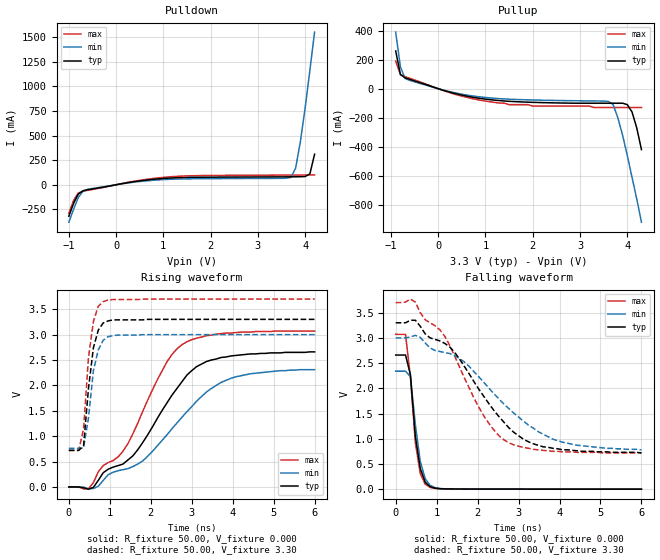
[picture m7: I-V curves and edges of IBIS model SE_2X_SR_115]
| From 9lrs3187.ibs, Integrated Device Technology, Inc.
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|   Model SE_2X_SR_115
[Model]   SE_2X_SR_115
Model_type   Output
Polarity   Inverting
Vmeas =   1.50V
Cref =   5.00pF
Rref =  50.000
Vref =   1.50V
C_comp   3.40pF   2.85pF   3.95pF
[Temperature Range]   27.00   70.00   0.000
[Voltage Range]   3.30V   3.00V   3.70V
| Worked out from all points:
|   slope of the pulldown table from 0 to 0.495 V, typ, clamps not added: 12.7 ohm
|   slope of the pullup table from 0 to 0.495 V, typ, clamps not added: 11.3 ohm
|   rising waveform, R_fixture 50.00, V_fixture 0.000: 20-80 % time 1.37ns typ, 1.63ns min, 1.16ns max; typ from 0 V to 2.66 V
|   rising waveform, R_fixture 50.00, V_fixture 3.30: 20-80 % time 210ps typ, 228ps min, 199ps max; typ from 0.72 V to 3.3 V
|   falling waveform, R_fixture 50.00, V_fixture 0.000: 20-80 % time 203ps typ, 224ps min, 214ps max; typ from 2.66 V to 0 V
|   falling waveform, R_fixture 50.00, V_fixture 3.30: 20-80 % time 1.38ns typ, 1.71ns min, 1.13ns max; typ from 3.3 V to 0.72 V
[Pulldown]
| voltage   I(typ)   I(min)   I(max)
|  -3.30   -4.16A   -4.01A   -4.26A
|  -3.10   -3.82A   -3.69A   -3.90A
|  -2.90   -3.48A   -3.37A   -3.55A
|  -2.70   -3.14A   -3.05A   -3.20A
|  -2.50   -2.80A   -2.72A   -2.85A
|  -2.30   -2.46A   -2.41A   -2.50A
|  -2.10   -2.12A   -2.09A   -2.15A
|  -1.90   -1.79A   -1.77A   -1.80A
|  -1.70   -1.45A   -1.45A   -1.45A
|  -1.50   -1.12A   -1.14A   -1.11A
-1V       -320mA     -380mA     -290mA
-900mV    -190mA     -250mA     -160mA
-800mV    -94.75mA   -130mA     -84.77mA
-700mV    -60.71mA   -64.75mA   -65.52mA
-600mV    -51.06mA   -45.2mA    -56.5mA
1.2V      69.5mA     56.57mA    82.87mA
3.7V      80.56mA    75.15mA    98.32mA
3.8V      80.96mA    170mA      98.58mA
3.9V      81.72mA    440mA      98.88mA
4V        83.73mA    780mA      99.22mA
4.1V      110mA      1.16A      99.62mA
4.2V      310mA      1.55A      100mA
|   4.30   0.66A   1.95A   0.10A
|   4.50   1.46A   2.77A   0.11A
|   4.70   2.32A   3.60A   0.58A
|   4.90   3.19A   4.43A   1.41A
|   5.10   4.07A   5.27A   2.30A
|   5.30   4.96A   6.12A   3.20A
|   5.50   5.85A   6.96A   4.12A
|   5.70   6.75A   7.81A   5.04A
|   5.90   7.65A   8.66A   5.97A
|   6.10   8.55A   9.52A   6.90A
|   6.60   10.81A   11.65A   9.23A
[Pullup]
| voltage   I(typ)   I(min)   I(max)
|  -3.30   10.68A   10.27A   10.94A
|  -3.10   9.79A   9.43A   10.01A
|  -2.90   8.89A   8.58A   9.09A
|  -2.70   7.99A   7.73A   8.16A
|  -2.50   7.10A   6.88A   7.23A
|  -2.30   6.20A   6.04A   6.31A
|  -2.10   5.31A   5.20A   5.38A
|  -1.90   4.43A   4.36A   4.47A
|  -1.70   3.54A   3.53A   3.55A
|  -1.50   2.67A   2.70A   2.64A
|  -1.00   0.59A   0.73A   0.50A
-900mV    260mA      390mA      190mA
-800mV    98.15mA    150mA      96.76mA
-700mV    74.35mA    69.94mA    82.79mA
-600mV    63.81mA    56.49mA    71.52mA
500mV     -44.25mA   -37.82mA   -51.47mA
1.5V      -86.95mA   -72.42mA   -110mA
3.5V      -100mA     -85.41mA   -130mA
3.7V      -100mA     -110mA     -130mA
3.9V      -100mA     -320mA     -130mA
4.1V      -160mA     -610mA     -130mA
4.2V      -270mA     -760mA     -130mA
4.3V      -420mA     -920mA     -130mA
|   4.50   -0.73A   -1.22A   -0.15A
|   4.70   -1.06A   -1.54A   -0.40A
|   4.90   -1.39A   -1.86A   -0.73A
|   5.10   -1.72A   -2.17A   -1.06A
|   5.30   -2.06A   -2.49A   -1.41A
|   5.50   -2.40A   -2.81A   -1.75A
|   5.70   -2.74A   -3.13A   -2.10A
|   5.90   -3.07A   -3.46A   -2.45A
|   6.10   -3.41A   -3.78A   -2.80A
|   6.60   -4.27A   -4.58A   -3.68A
[Ramp]
| variable   typ   min   max
dV/dt_r   1.59/1.36n   1.39/1.64n   1.84/1.15n
dV/dt_f   1.55/1.38n   1.33/1.70n   1.79/1.13n
R_load = 50.00
[Rising Waveform]
R_fixture = 50.00
V_fixture = 0.000
V_fixture_min = 0.000
V_fixture_max = 0.000
| time   V(typ)   V(min)   V(max)
0s        0V         1.34uV     0V
480ps     -43.33mV   -36.21mV   -37.06mV
840ps     280mV      130mV      420mV
1.32ns    450mV      340mV      700mV
1.8ns     870mV      510mV      1.48V
2.4ns     1.66V      1.03V      2.47V
2.76ns    2.07V      1.37V      2.8V
3.12ns    2.37V      1.69V      2.93V
3.96ns    2.58V      2.14V      3.03V
6ns       2.66V      2.31V      3.07V
[Rising Waveform]
R_fixture = 50.00
V_fixture = 3.30
V_fixture_min = 3.00
V_fixture_max = 3.70
| time   V(typ)   V(min)   V(max)
0s        720mV      760mV      720mV
240ps     720mV      760mV      720mV
360ps     810mV      770mV      1.14V
480ps     1.94V      1.36V      2.55V
600ps     2.74V      2.29V      3.26V
720ps     3.09V      2.7V       3.56V
840ps     3.23V      2.89V      3.65V
960ps     3.27V      2.96V      3.68V
1.2ns     3.29V      2.99V      3.69V
6ns       3.3V       3V         3.7V
[Falling Waveform]
R_fixture = 50.00
V_fixture = 0.000
V_fixture_min = 0.000
V_fixture_max = 0.000
| time   V(typ)   V(min)   V(max)
0s        2.66V      2.34V      3.07V
240ps     2.66V      2.34V      3.07V
360ps     2.27V      2.23V      2.22V
480ps     1.05V      1.28V      920mV
600ps     410mV      550mV      310mV
720ps     140mV      210mV      100mV
840ps     48.93mV    76.66mV    35.05mV
960ps     19.96mV    29.7mV     15.02mV
1.32ns    4.41mV     4.54mV     4.01mV
6ns       49.61uV    110uV      21.14uV
[Falling Waveform]
R_fixture = 50.00
V_fixture = 3.30
V_fixture_min = 3.00
V_fixture_max = 3.70
| time   V(typ)   V(min)   V(max)
0s        3.3V       3V         3.7V
360ps     3.35V      3.02V      3.77V
720ps     3.08V      2.9V       3.36V
1.08ns    2.94V      2.73V      3.16V
1.44ns    2.71V      2.65V      2.64V
2.16ns    1.83V      2.11V      1.44V
2.76ns    1.22V      1.6V       920mV
3.24ns    940mV      1.27V      810mV
3.84ns    810mV      990mV      750mV
6ns       720mV      780mV      720mV
